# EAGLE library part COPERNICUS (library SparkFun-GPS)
Trimble Copernicus II GPS Receiver The Trimble Copernicus II delivers proven performance and Trimble quality for a new generation of position-enabled products. It features the TrimCore™ navigation software for extremely fast startup times and high performance in foliage canopy and urban canyon environments. SparkFun Products GPS Module - Copernicus II (12 Channel) (GPS-10922) SparkFun GPS Module - Copernicus II DIP (12 Channel) (GPS-11858)
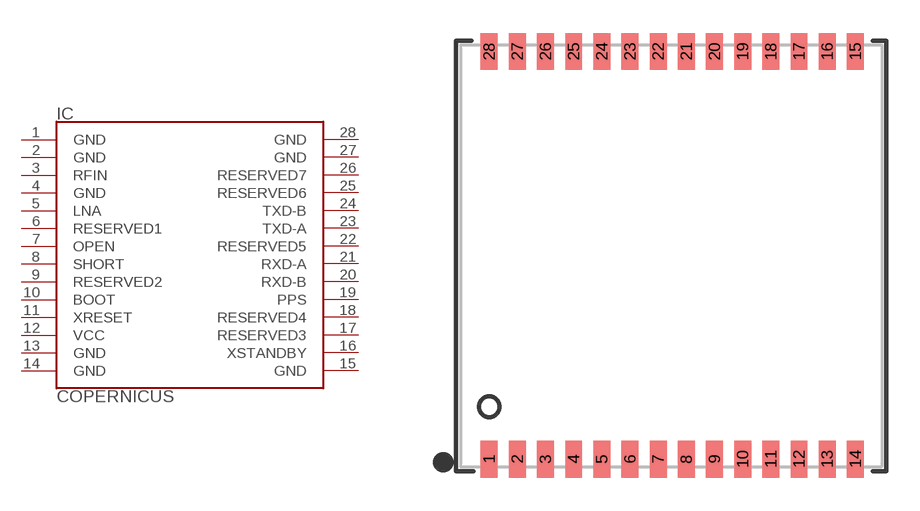
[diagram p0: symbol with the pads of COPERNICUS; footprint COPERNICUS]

Designator prefix IC

## COPERNICUSSMD (PROD_ID: GPS-10735; SF_ID: GPS-10922)  [COPERNICUS]
1  GND
2  GND
3  RFIN
4  GND
5  LNA
6  RESERVED1
7  OPEN
8  SHORT
9  RESERVED2
10  BOOT
11  XRESET
12  VCC
13  GND
14  GND
15  GND
16  XSTANDBY
17  RESERVED3
18  RESERVED4
19  PPS
20  RXD-B
21  RXD-A
22  RESERVED5
23  TXD-A
24  TXD-B
25  RESERVED6
26  RESERVED7
27  GND
28  GND

## Footprint COPERNICUS (pad centres in mm)
Trimble Copernicus and Copernicus II GPS Receiver Datasheet
smd 0.762 x 1.651: 1 -8.2,-9.164; 2 -6.93,-9.164; 3 -5.66,-9.164; 4 -4.39,-9.164; 5 -3.12,-9.164; 6 -1.85,-9.164; 7 -0.58,-9.164; 8 0.69,-9.164; 9 1.96,-9.164; 10 3.23,-9.164; 11 4.5,-9.164; 12 5.77,-9.164; 13 7.04,-9.164; 14 8.31,-9.164; 15 8.31,9.2; 16 7.04,9.2; 17 5.77,9.2; 18 4.5,9.2; 19 3.23,9.2; 20 1.96,9.2; 21 0.69,9.2; 22 -0.58,9.2; 23 -1.85,9.2; 24 -3.12,9.2; 25 -4.39,9.2; 26 -5.66,9.2; 27 -6.93,9.2; 28 -8.2,9.2

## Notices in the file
Licensing: Creative Commons ShareAlike 4.0 International - https://creativecommons.org/licenses/by-sa/4.0
